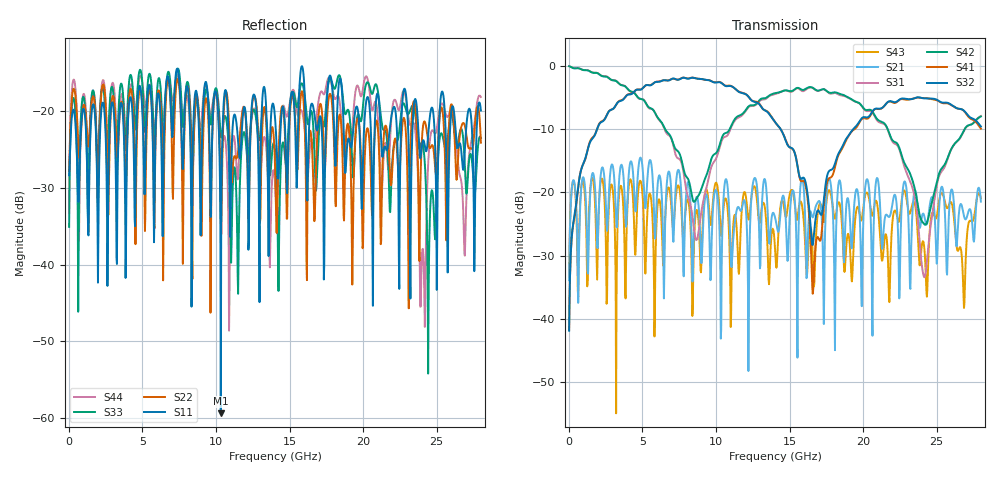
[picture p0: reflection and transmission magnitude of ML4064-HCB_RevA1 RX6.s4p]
! TOUCHSTONE file generated by CST DESIGN STUDIO
! Date and time: Wed Aug 26 10:43:56 2020
! Project name:  Project name: C:\Users\Simulation2\Temp\DE66\Untitled_0.cst
! Tree item: Tasks\SPara1\S-Parameters
# GHz S MA R 50
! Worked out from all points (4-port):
!   1000 points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, 28 MHz to 28 GHz, reference 50 ohm
!   strongest paths, dB at 28 MHz, 7.028 GHz, 14.03 GHz, 21.03 GHz, 28 GHz:
!     S32: -41.9, -2.0, -8.9, -6.8, -9.6
!     S41: -41.7, -2.1, -8.9, -6.8, -9.9
!     S42: -0.1, -11.8, -4.3, -8.6, -8.0
!     S31: -0.1, -11.9, -4.5, -8.8, -7.9
!     S21: -33.9, -23.2, -24.1, -18.3, -21.5
!     S43: -33.3, -24.3, -29.4, -23.1, -21.0
!   lowest |S11| = -59.3 dB at 10.33 GHz (marker M1), VSWR 1.00, Z = 50 + j0.0978 ohm
!   |S11| at or under -10 dB: start of sweep to end of sweep
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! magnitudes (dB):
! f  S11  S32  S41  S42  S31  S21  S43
! 28 MHz  -28.4  -41.9  -41.7  -0.1  -0.1  -33.9  -33.3
! 2.1 GHz  -24.5  -9.1  -9.1  -1.4  -1.4  -19.6  -20.1
! 10.33 GHz  -59.3  -2.7  -2.6  -11.9  -12.3  -43.1  -26.4
! 16.6 GHz  -19.4  -28.0  -35.5  -3.5  -3.6  -23.9  -31.6
! 22.79 GHz  -17.1  -5.2  -5.3  -15.3  -15.9  -18.3  -19.7
! 24.16 GHz  -24.2  -5.2  -5.1  -25.0  -33.4  -23.8  -29.0
! 28 GHz  -19.9  -9.6  -9.9  -8.0  -7.9  -21.5  -21.0
